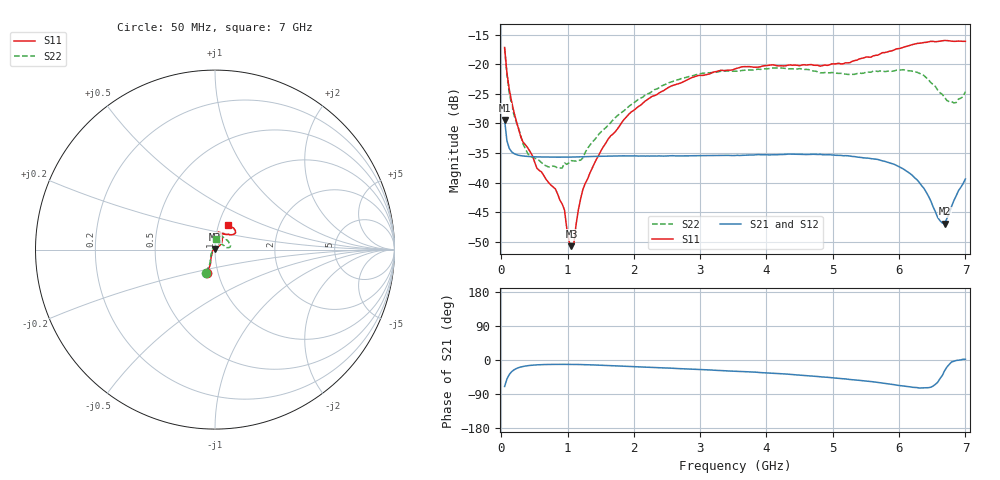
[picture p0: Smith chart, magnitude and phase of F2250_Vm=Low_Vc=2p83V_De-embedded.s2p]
! Integrated Device Technology
! Corporate Headquarters
! 6024 Silver Creek Valley Road
! San Jose, CA 95138  USA
! Phone:  1-408-284-8200
! Toll Free:  1-800-223-1366
! Webpage:  http://www.idt.com/
! Timing and RF Division
! 515 Groton Road, Suite 102
! Westford, MA 01886-6024
! Device:  F2250
! Description: Voltage Variable RF Attenuator
! Frequency:  50.0 -  6000.00 MHz
! Package:  3x3 mm Thin QFN Plastic Package: 16 pin
! Ports:  2 RF, 3 DC
!  Pin  1  = GND
!  Pin  2  = NC
!  Pin  3  = RF1  = Port 1
!  Pin  4  = NC
!  Pin  5  = GND
!  Pin  6  = GND
!  Pin  7  = GND
!  Pin  8  = GND
!  Pin  9  = NC
!  Pin 10  = RF2  = Port 2
!  Pin 11  = NC
!  Pin 12  = GND
!  Pin 13  = GND
!  Pin 14  = VCNTRL
!  Pin 15  = VDD
!  Pin 16  = VMODE
! Vcntrl:  2.830 Volts
! Vmode:  +0.000 Volts
! Vdd:  +3.30  Volts
! Current:  1.174 mA
! Data:  The device was measured on a the F2250 evaluation board which has
!  individual transmission lines to the RF pins.  Data was collected
!  using a calibrated network analyzer.  The evaluation board was
!  de-embedded using a TRL calibration technique.
!  The reference plane is the edge of the package pin.
! Misc:  SN 10
!  Action Tracker AT0258
! Date Measured:  2014-11-26
! Date:  2015-10-15  MJV
! Note:
!  Integrated Device Technology supplies this data as a sample of measured
!  data at the package pin for this product.  Your particular data for this
!  product may vary.
!  Data was taken at 25 degrees C.
!  Integrated Device Technology reserves the right to change this data at anytime.
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# GHz S dB R 50
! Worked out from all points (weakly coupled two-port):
!   201 points, 50 MHz to 7 GHz, reference 50 ohm
!   highest |S21| = -29.42 dB at 50 MHz (marker M1); lowest = -46.9 dB at 6.687 GHz (marker M2)
!   lowest |S11| = -50.7 dB at 1.058 GHz (marker M3), VSWR 1.01, Z = 49.8 + j0.24 ohm
!   |S11| at or under -10 dB: start of sweep to end of sweep
!   |S22| runs from -37.5 to -17.3 dB; largest |S21 - S12| = 6.3e-05
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0.05  -17.18 -108.6  -29.42 -69.8  -29.41 -69.8  -17.28 -111.0
0.08475  -21.45 -107.4  -32.92 -50.3  -32.92 -50.3  -21.75 -110.2
0.15425  -26.23 -116.6  -34.76 -31.2  -34.75 -31.1  -26.81 -122.4
0.29325  -32.21 -127.9  -35.43 -18.5  -35.43 -18.5  -32.10 -137.5
0.3975  -34.09 -141.8  -35.56 -15.0  -35.56 -15.0  -35.05 -160.6
0.91875  -43.58 157.8  -35.68 -11.5  -35.69 -11.5  -37.52 133.5
0.9535  -44.62 170.0  -35.69 -11.5  -35.69 -11.5  -36.67 131.3
1.023  -49.94 144.2  -35.67 -11.6  -35.68 -11.6  -36.63 115.8
1.05775  -50.70 124.2  -35.67 -11.6  -35.67 -11.6  -36.27 110.9
1.0925  -50.44 90.1  -35.66 -11.7  -35.66 -11.7  -36.32 106.3
1.162  -44.62 57.1  -35.64 -11.9  -35.64 -11.9  -36.23 95.6
1.2315  -41.11 44.3  -35.61 -12.1  -35.61 -12.1  -35.78 85.9
1.6485  -32.10 42.0  -35.52 -14.6  -35.52 -14.6  -29.88 64.6
1.96125  -28.05 42.2  -35.46 -17.2  -35.46 -17.2  -26.80 56.8
2.37825  -24.87 47.3  -35.48 -20.3  -35.48 -20.3  -23.99 56.8
3.525  -20.79 72.5  -35.40 -29.5  -35.40 -29.6  -21.18 74.7
4.7065  -20.17 72.4  -35.20 -42.6  -35.19 -42.6  -21.14 72.2
5.85325  -17.81 40.5  -36.64 -63.4  -36.63 -63.4  -21.14 23.0
6.27025  -16.50 40.0  -39.50 -72.8  -39.50 -72.8  -21.36 9.7
6.68725  -15.99 48.7  -46.89 -28.0  -46.87 -27.4  -25.63 28.6
6.861  -16.13 55.1  -42.21 -1.3  -42.16 -1.4  -26.46 58.0
7  -16.13 63.2  -39.36 1.9  -39.33 1.7  -24.63 83.1
